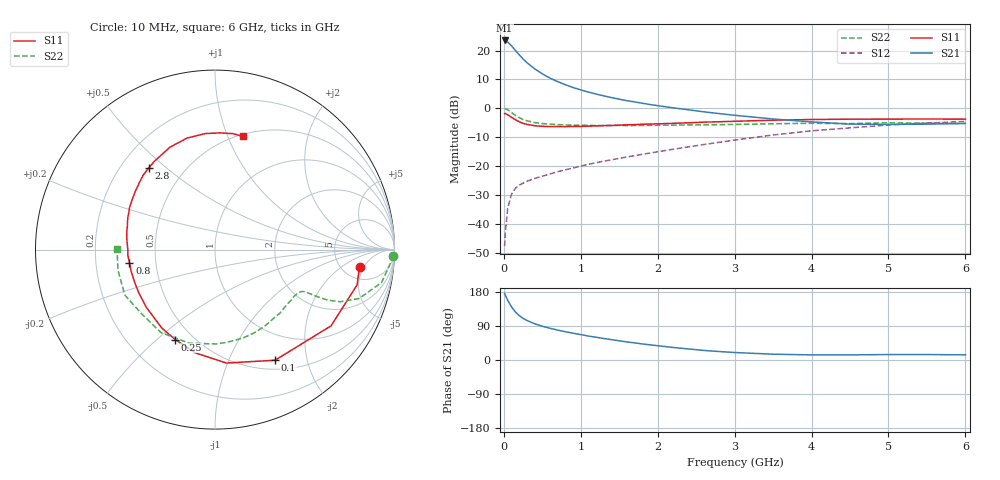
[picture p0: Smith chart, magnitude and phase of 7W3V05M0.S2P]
! Infineon Technologies  Discrete & RF Semiconductors
! BFS17W
! Si NPN RF Bipolar Junction Transistor in SOT323
! VCE = 3 V  IC = 5 mA
! Common Emitter S-Parameters:  August  1999
# GHz  S  MA  R  50
!  f  S11  S21  S12  S22
! GHz  MAG  ANG  MAG  ANG  MAG  ANG  MAG  ANG
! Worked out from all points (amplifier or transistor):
!   36 points, 10 MHz to 6 GHz, reference 50 ohm
!   highest |S21| = 23.5 dB at 10 MHz (marker M1)
!   |S21| within 3 dB of that: start of sweep to 136.1 MHz
!   unconditionally stable (mu >= 1): 548.3 MHz to 2.906 GHz; 4.204 GHz to end of sweep
!   at 250 MHz: K = 0.59, MSG = 21.5 dB, |S12| = -25.9 dB
!   at 1.4 GHz: K = 1.25, MAG = 7.7 dB, |S12| = -17.8 dB
!   at 6 GHz: K = 1.08, MAG = -2.1 dB, |S12| = -4.5 dB
!   S11 on the Smith chart (normalised r, x): 10 MHz: 7.31, -4.04; 100 MHz: 0.62, -1.50; 250 MHz: 0.40, -0.58; 800 MHz: 0.35, -0.07; 2.8 GHz: 0.32, +0.44; 6 GHz: 0.52, +1.14
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0.01  0.8108 -6.7  14.98 176.0  0.0041 81.5  0.9942 -1.9
0.02  0.8159 -13.9  14.92 170.8  0.0073 84.0  0.9794 -4.6
0.05  0.7737 -33.3  14.13 157.7  0.0185 73.0  0.946 -11.2
0.1  0.7013 -61.5  12.08 140.1  0.0327 61.5  0.8484 -18.7
0.15  0.6353 -84.2  10.09 126.6  0.0413 54.2  0.756 -22.6
0.2  0.5858 -100.8  8.454 117.2  0.0467 50.6  0.69 -24.1
0.25  0.5479 -113.8  7.172 110.0  0.0507 48.5  0.6403 -24.6
0.3  0.5281 -124.1  6.192 104.4  0.0546 48.3  0.6091 -24.8
0.4  0.5 -139.9  4.843 95.6  0.061 48.6  0.5663 -25.0
0.5  0.4879 -150.8  3.959 89.1  0.0669 50.1  0.5454 -25.3
0.6  0.4829 -159.1  3.336 83.7  0.073 51.7  0.5319 -26.2
0.8  0.4819 -171.4  2.563 74.6  0.0862 55.3  0.5155 -29.3
0.9  0.4868 -176.2  2.295 70.7  0.0926 56.6  0.5108 -31.0
1.1  0.4915 175.4  1.912 63.2  0.1075 58.7  0.5067 -35.2
1.3  0.5017 168.3  1.643 56.7  0.1217 60.4  0.5033 -40.1
1.6  0.5187 159.3  1.358 47.7  0.1437 62.4  0.5025 -47.7
2.2  0.5499 143.8  1.021 33.1  0.1957 64.7  0.5125 -65.0
2.8  0.5858 129.1  0.811 22.3  0.2578 63.8  0.521 -83.5
3.5  0.6236 113.7  0.654 15.3  0.3456 59.4  0.5408 -105.6
4.5  0.6487 94.8  0.533 13.5  0.459 47.4  0.5435 -139.0
5.5  0.6538 81.2  0.532 14.4  0.5555 35.0  0.5527 -168.0
6  0.6495 76.1  0.548 13.6  0.5925 28.9  0.5463 179.4
